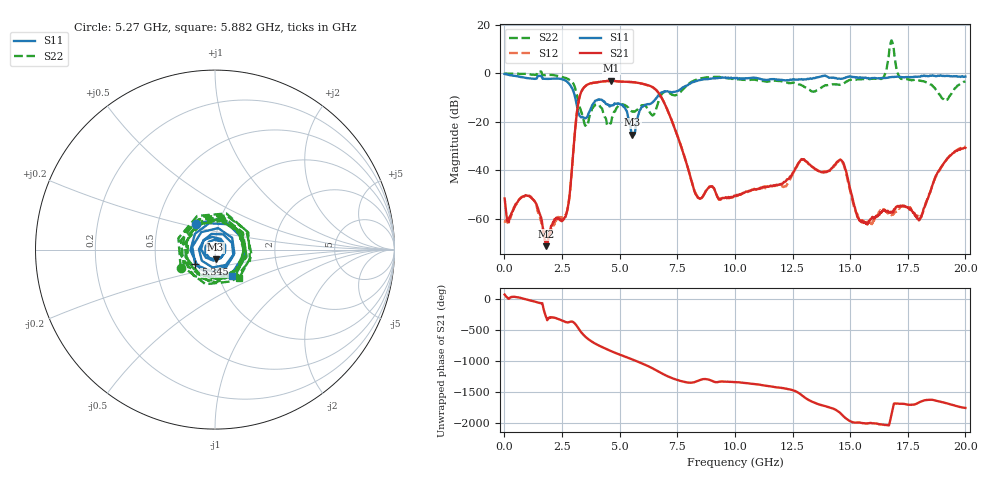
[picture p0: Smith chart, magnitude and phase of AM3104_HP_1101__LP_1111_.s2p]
!Created with skrf (http://scikit-rf.org).
# Hz S RI R 50.0
!freq ReS11 ImS11 ReS21 ImS21 ReS12 ImS12 ReS22 ImS22
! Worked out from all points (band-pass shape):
!   1601 points, 10 MHz to 20 GHz, reference 50 ohm
!   highest |S21| = -3.04 dB at 4.633 GHz (marker M1); lowest = -71.2 dB at 1.809 GHz (marker M2)
!   |S21| within 3 dB of the highest: 3.43 GHz to 6.486 GHz (3.056 GHz wide, 61.6 % of centre)
!   lowest |S11| = -25.3 dB at 5.545 GHz (marker M3), VSWR 1.12, Z = 50 - j5.47 ohm
!   |S11| at or under -10 dB: 3.072 GHz to 6.609 GHz (3.537 GHz wide, 73.1 % of centre)
!   |S22| runs from -21.8 to 13.6 dB; largest |S21 - S12| = 0.081
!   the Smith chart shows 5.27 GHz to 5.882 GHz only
!   S11 on the Smith chart (normalised r, x): 5.27 GHz: 0.78, +0.23; 5.345 GHz: 0.79, -0.13; 5.882 GHz: 1.15, -0.35
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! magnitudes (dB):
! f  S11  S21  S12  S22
! 10 MHz  -0.2  -51.6  -61.0  0.0
! 197.4 MHz  -0.7  -61.4  -61.0  -0.1
! 1.084 GHz  -2.0  -50.7  -50.4  -0.4
! 1.809 GHz  -2.3  -71.2  -69.6  -0.7
! 2.721 GHz  -3.4  -56.8  -56.6  -2.1
! 3.346 GHz  -18.1  -7.4  -7.4  -16.0
! 4.633 GHz  -13.2  -3.0  -3.2  -20.2
! 5.27 GHz  -15.0  -3.4  -3.5  -13.3
! 5.345 GHz  -17.3  -3.4  -3.5  -13.9
! 5.545 GHz  -25.3  -3.5  -3.6  -15.6
! 5.882 GHz  -15.2  -4.0  -4.0  -13.7
! 6.682 GHz  -9.0  -7.9  -7.9  -11.5
! 8.368 GHz  -3.0  -50.9  -50.6  -2.3
! 10.01 GHz  -2.0  -50.5  -50.8  -2.4
! 13.34 GHz  -2.2  -38.5  -38.4  -7.4
! 14.64 GHz  -2.1  -36.0  -36.4  -4.6
! 15.49 GHz  -1.8  -61.4  -60.8  -2.4
! 16.4 GHz  -1.9  -56.8  -56.0  -1.9
! 16.68 GHz  -1.7  -57.1  -58.2  7.3
! 18.01 GHz  -1.4  -60.1  -59.1  -3.0
! 19.14 GHz  -1.1  -36.1  -36.1  -11.2
! 20 GHz  -1.3  -30.7  -30.2  -3.3
